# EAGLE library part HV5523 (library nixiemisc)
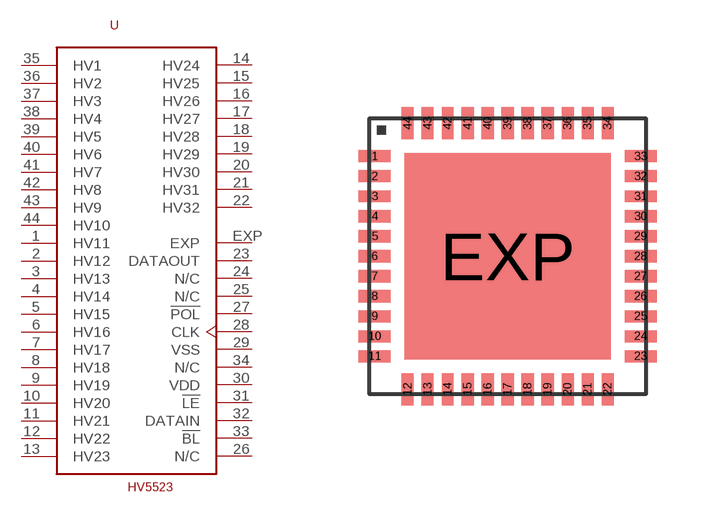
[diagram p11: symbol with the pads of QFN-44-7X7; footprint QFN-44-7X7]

Designator prefix U

## HV5523  [QFN-44-7X7]
1  HV11  pas
2  HV12  pas
3  HV13  pas
4  HV14  pas
5  HV15  pas
6  HV16  pas
7  HV17  pas
8  HV18  pas
9  HV19  pas
10  HV20  pas
11  HV21  pas
12  HV22  pas
13  HV23  pas
14  HV24  pas
15  HV25  pas
16  HV26  pas
17  HV27  pas
18  HV28  pas
19  HV29  pas
20  HV30  pas
21  HV31  pas
22  HV32  pas
23  DATAOUT
24  N/C  nc
25  N/C  nc
26  N/C  nc
27  !POL  pas
28  CLK  pas
29  VSS  pwr
30  VDD  pwr
31  !LE  pas
32  DATAIN
33  !BL  pas
34  N/C  nc
35  HV1  pas
36  HV2  pas
37  HV3  pas
38  HV4  pas
39  HV5  pas
40  HV6  pas
41  HV7  pas
42  HV8  pas
43  HV9  pas
44  HV10  pas
EXP  EXP  pwr

## Footprint QFN-44-7X7 (pad centres in mm)
QFN-44 (7x7x1.8mm) Source: http://www.st.com/stonline/products/literature/ds/11020.pdf
smd 0.8 x 0.3: 1 -3.325,2.5; 2 -3.325,2; 3 -3.325,1.5; 4 -3.325,1; 5 -3.325,0.5; 6 -3.325,0; 7 -3.325,-0.5; 8 -3.325,-1; 9 -3.325,-1.5; 10 -3.325,-2; 11 -3.325,-2.5; 23 3.325,-2.5; 24 3.325,-2; 25 3.325,-1.5; 26 3.325,-1; 27 3.325,-0.5; 28 3.325,0; 29 3.325,0.5; 30 3.325,1; 31 3.325,1.5; 32 3.325,2; 33 3.325,2.5
smd 0.3 x 0.8: 12 -2.5,-3.325; 13 -2,-3.325; 14 -1.5,-3.325; 15 -1,-3.325; 16 -0.5,-3.325; 17 0,-3.325; 18 0.5,-3.325; 19 1,-3.325; 20 1.5,-3.325; 21 2,-3.325; 22 2.5,-3.325; 34 2.5,3.325; 35 2,3.325; 36 1.5,3.325; 37 1,3.325; 38 0.5,3.325; 39 0,3.325; 40 -0.5,3.325; 41 -1,3.325; 42 -1.5,3.325; 43 -2,3.325; 44 -2.5,3.325
smd 5.15 x 5.15: EXP 0,0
